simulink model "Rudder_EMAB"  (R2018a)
settings: Solver=ode45  StartTime=0.0  StopTime=1  RelTol=1e-3  EnableMultiTasking=on
InitFcn:
  | init
StopFcn:
  | pl
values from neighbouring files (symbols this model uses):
  Be = 25    [init.m]
  d2r = pi/180    (= 0.0174532925199)    [init.m]
  Ja = 2.0e-4    (= 0.0002)    [init.m]
  Je = 2.2    [init.m]
  Jm = 5.0e-5    (= 5e-05)    [init.m]
  Kdmp = 0.001    [init.m]
  Keff = 0.85    [init.m]
  Kgs = 400.0    (= 400)    [init.m]
  Ki = 5.0    (= 5)    [init.m]
  Kl = 12/Kli    (= 1800000)    [init.m]
  Kmfr = 0.03    [init.m]
  Kp = 140    [init.m]
  Krfb = 0.0005    [init.m]
  Kt = 12/Kti    (= 1674418.60465)    [init.m]
  Kv = 260    [init.m]
  Ngear = 10.2    [init.m]
  Nscrew = 0.0026    [init.m]
  R = 0.287    [init.m]    (also in lqr_des.m = diag(R))
  Vlim = 100    [init.m]
  Wmb = 1500    [init.m]
undefined symbols (not defined in the file or in its folder): coulomb

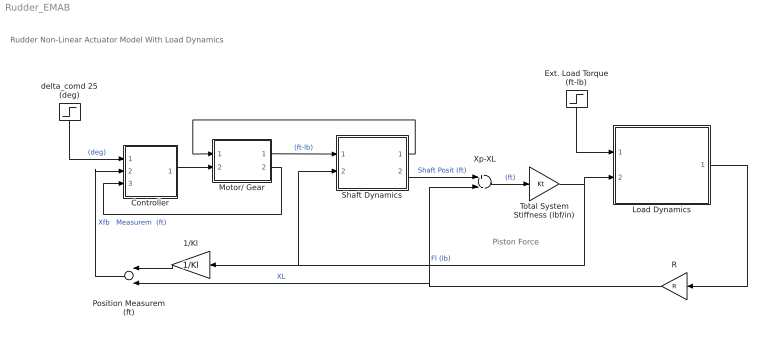
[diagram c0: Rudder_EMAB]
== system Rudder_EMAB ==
  note: Piston Force
  note: Rudder Non-Linear Actuator Model With Load Dynamics
  1/Kl : Gain  Gain=1/Kl
  Controller : Subsystem
  Ext. Load Torque (ft-lb) : Step  Time=0  After=0  SampleTime=0
  Load Dynamics : Subsystem
  Motor/ Gear : Subsystem
  Position Measurem (ft) : Sum
  R : Gain  Gain=R
  Shaft Dynamics : Subsystem
  Total System Stiffness (lbf/in) : Gain  Gain=Kt
  Xp-XL : Sum  Inputs=+-
  delta_comd 25 (deg) : Step  Time=0  After=25  SampleTime=0
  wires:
  Shaft Dynamics/2(Xp) -> Xp-XL/1  "Shaft Posit (ft)"
  Xp-XL/1 -> Total System Stiffness (lbf/in)/1  "(ft)"
  Total System Stiffness (lbf/in)/1 -> Load Dynamics/2(FL), Shaft Dynamics/2(FL), 1/Kl/1  "Fl (lb)"
  1/Kl/1 -> Position Measurem (ft)/1
  Controller/1(V) -> Motor/ Gear/2(Vin)
  Motor/ Gear/1(Tm) -> Shaft Dynamics/1(Tq-mot)  "(ft-lb)"
  Load Dynamics/1(Delta (rad)) -> R/1
  Position Measurem (ft)/1 -> Controller/2(Xp-fb)  "Xfb   Measurem  (ft)"
  Shaft Dynamics/1(Xp-dot) -> Motor/ Gear/1(Xp-dot)
  R/1 -> Position Measurem (ft)/2, Xp-XL/2  "XL"
  Motor/ Gear/2(mr) -> Controller/3(rotor)
  delta_comd 25 (deg)/1 -> Controller/1(delt-cmd)  "(deg)"
  Ext. Load Torque (ft-lb)/1 -> Load Dynamics/1(Load-Torque)

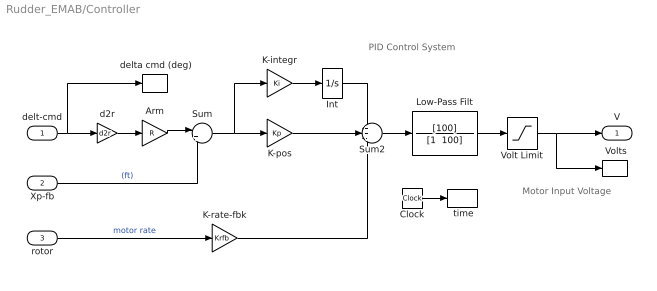
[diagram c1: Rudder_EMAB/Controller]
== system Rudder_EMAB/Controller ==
  note: PID Control System
  note: Motor Input Voltage
  delt-cmd : Inport
  Xp-fb : Inport  Port=2
  rotor : Inport  Port=3
  " Volts" : ToWorkspace  VariableName=V  SampleTime=-1
  " delta cmd (deg)" : ToWorkspace  VariableName=delc  SampleTime=-1
  " time" : ToWorkspace  VariableName=time  SampleTime=-1
  Arm : Gain  Gain=R
  Clock : Clock
  Int : Integrator  UpperSaturationLimit=1  LowerSaturationLimit=-1
  K-integr : Gain  Gain=Ki
  K-pos : Gain  Gain=Kp
  K-rate-fbk : Gain  Gain=Krfb
  Low-Pass Filt : TransferFcn  Numerator=[100]  Denominator="[1  100]"
  Sum : Sum  Inputs=|+-
  Sum2 : Sum  Inputs=++-
  Volt Limit : Saturate  UpperLimit=Vlim  LowerLimit=-Vlim
  d2r : Gain  Gain=d2r
  V : Outport
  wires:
  Low-Pass Filt/1 -> Volt Limit/1
  delt-cmd/1 -> " delta cmd (deg)"/1, d2r/1
  Xp-fb/1 -> Sum/2  "(ft)"
  Sum/1 -> K-pos/1, K-integr/1
  rotor/1 -> K-rate-fbk/1  "motor rate"
  Sum2/1 -> Low-Pass Filt/1
  K-pos/1 -> Sum2/2
  Volt Limit/1 -> V/1, " Volts"/1
  Clock/1 -> " time"/1
  K-integr/1 -> Int/1
  Int/1 -> Sum2/1
  K-rate-fbk/1 -> Sum2/3
  Arm/1 -> Sum/1
  d2r/1 -> Arm/1

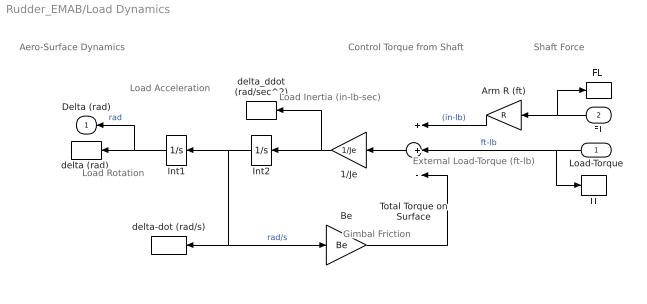
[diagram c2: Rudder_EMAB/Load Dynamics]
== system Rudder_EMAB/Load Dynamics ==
  note: Aero-Surface Dynamics
  note: Load Acceleration
  note: Gimbal Friction
  note: External Load-Torque (ft-lb)
  note: Control Torque from Shaft
  note: Shaft Force
  note: Load Inertia (in-lb-sec)
  note: Load Rotation
  Load-Torque : Inport
  FL : Inport  Port=2
  1/Je : Gain  Gain=1/Je
  Arm R (ft) : Gain  Gain=R
  Be : Gain  Gain=Be
  "FL " : ToWorkspace  VariableName=FL  SampleTime=-1
  Int1 : Integrator
  Int2 : Integrator
  TL : ToWorkspace  VariableName=TL  SampleTime=-1
  Total Torque on Surface : Sum  Inputs=++-
  "delta (rad) " : ToWorkspace  VariableName=delta  SampleTime=-1
  delta-dot (rad/s) : ToWorkspace  VariableName=deldot  SampleTime=-1
  delta_ddot (rad/sec^2) : ToWorkspace  VariableName=deldd  SampleTime=-1
  Delta (rad) : Outport
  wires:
  Arm R (ft)/1 -> Total Torque on Surface/1  "(in-lb)"
  Total Torque on Surface/1 -> 1/Je/1
  Int1/1 -> "delta (rad) "/1, Delta (rad)/1  "rad"
  Load-Torque/1 -> Total Torque on Surface/2, TL/1  "ft-lb"
  FL/1 -> "FL "/1, Arm R (ft)/1
  Int2/1 -> Int1/1, Be/1, delta-dot (rad/s)/1  "rad/s"
  1/Je/1 -> Int2/1, delta_ddot (rad/sec^2)/1
  Be/1 -> Total Torque on Surface/3

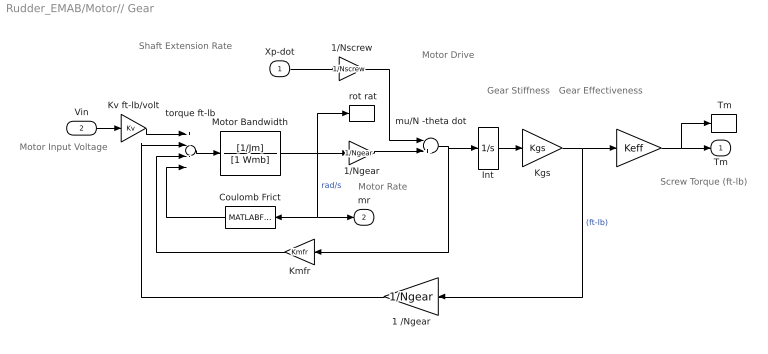
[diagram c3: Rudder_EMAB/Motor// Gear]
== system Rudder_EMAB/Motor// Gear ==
  note: Gear Effectiveness
  note: Gear Stiffness
  note: Motor Drive
  note: Shaft Extension Rate
  note: Motor Rate
  note: Motor Input Voltage
  note: Screw Torque (ft-lb)
  Xp-dot : Inport
  Vin : Inport  Port=2
  " " : Gain  Gain=Keff
  " Tm" : ToWorkspace  VariableName=Tm  SampleTime=-1
  " rot rat" : ToWorkspace  VariableName=mrat  SampleTime=-1
  1 /Ngear : Gain  Gain=1/Ngear
  1/Ngear : Gain  Gain=1/Ngear
  1/Nscrew : Gain  Gain=1/Nscrew
  Coulomb Frict : MATLABFcn  MATLABFcn=coulomb(0.0037, u(1) )
  Int : Integrator  LimitOutput=on  UpperSaturationLimit=0.4  LowerSaturationLimit=-0.4
  Kgs : Gain  Gain=Kgs
  Kmfr : Gain  Gain=Kmfr
  Kv ft-lb/volt : Gain  Gain=Kv
  Motor Bandwidth : TransferFcn  Numerator=[1/Jm]  Denominator=[1 Wmb]
  mu/N -theta dot : Sum  Inputs=-+
  torque ft-lb : Sum  Inputs=+---
  Tm : Outport
  mr : Outport  Port=2
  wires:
  mu/N -theta dot/1 -> Int/1, Kmfr/1
  torque ft-lb/1 -> Motor Bandwidth/1
  1 /Ngear/1 -> torque ft-lb/2
  Motor Bandwidth/1 -> 1/Ngear/1, " rot rat"/1, mr/1, Coulomb Frict/1  "rad/s"
  1/Ngear/1 -> mu/N -theta dot/2
  Kgs/1 -> 1 /Ngear/1, " "/1  "(ft-lb)"
  Xp-dot/1 -> 1/Nscrew/1
  Vin/1 -> Kv ft-lb/volt/1
  " "/1 -> Tm/1, " Tm"/1
  Kv ft-lb/volt/1 -> torque ft-lb/1
  1/Nscrew/1 -> mu/N -theta dot/1
  Kmfr/1 -> torque ft-lb/3
  Int/1 -> Kgs/1
  Coulomb Frict/1 -> torque ft-lb/4

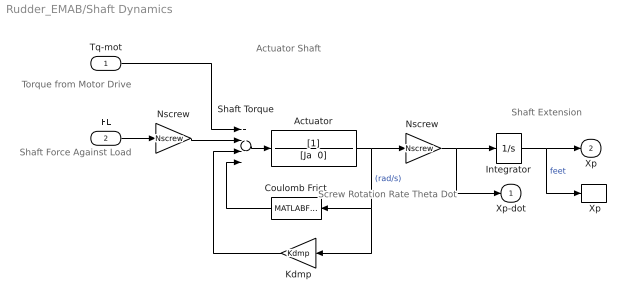
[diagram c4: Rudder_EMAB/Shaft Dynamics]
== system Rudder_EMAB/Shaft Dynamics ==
  note: Actuator Shaft
  note: Torque from Motor Drive
  note: Shaft Force Against Load
  note: Screw Rotation Rate Theta Dot
  note: Shaft Extension
  Tq-mot : Inport
  FL : Inport  Port=2
  " Xp" : ToWorkspace  VariableName=Xp  SampleTime=-1
  Actuator : TransferFcn  Denominator="[Ja  0]"
  Coulomb Frict : MATLABFcn  MATLABFcn=coulomb(0.1, u(1) )
  Integrator : Integrator
  Kdmp : Gain  Gain=Kdmp
  Nscrew : Gain  Gain=Nscrew
  "Nscrew " : Gain  Gain=Nscrew
  Shaft Torque : Sum  Inputs=+---
  Xp-dot : Outport
  Xp : Outport  Port=2
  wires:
  Actuator/1 -> "Nscrew "/1, Coulomb Frict/1, Kdmp/1  "(rad/s)"
  Shaft Torque/1 -> Actuator/1
  Tq-mot/1 -> Shaft Torque/1
  Integrator/1 -> Xp/1, " Xp"/1  "feet"
  FL/1 -> Nscrew/1
  Nscrew/1 -> Shaft Torque/2
  "Nscrew "/1 -> Integrator/1, Xp-dot/1
  Kdmp/1 -> Shaft Torque/3
  Coulomb Frict/1 -> Shaft Torque/4
